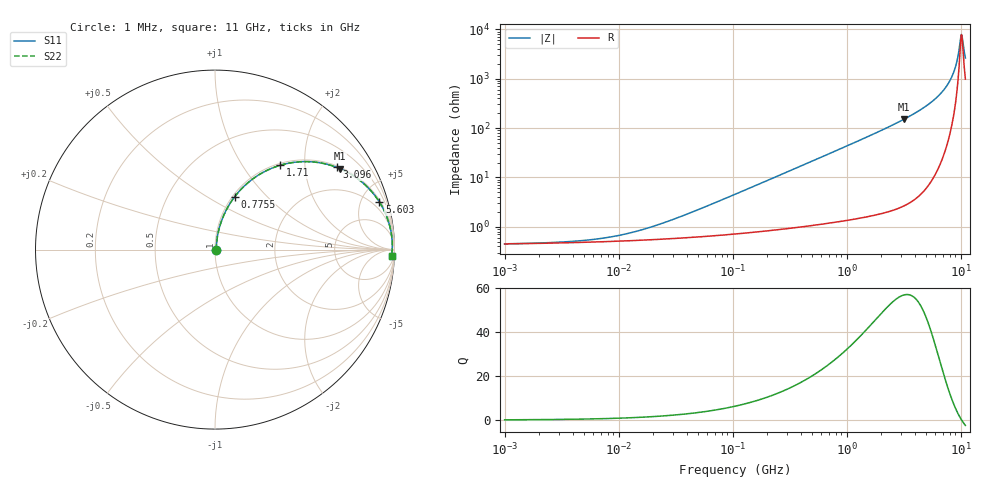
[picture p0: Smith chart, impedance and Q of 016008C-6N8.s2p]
# MHz S MA R 50
!Freq  MagS11  AngS11  MagS21  AngS21  MagS12  AngS12  MagS22  AngS22
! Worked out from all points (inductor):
!   801 points, 1 MHz to 11 GHz, reference 50 ohm
!   read as one part in series: L = 6.8 nH near 42.83 MHz
!   highest Q = 57.1 at 3.206 GHz (marker M1), where L = 7.55 nH
!   self-resonance near 10.14 GHz
!   S11 on the Smith chart (normalised r, x): 1 MHz: 1.01, +0.00; 775.5 MHz: 1.02, +0.67; 1.71 GHz: 1.03, +1.50; 3.096 GHz: 1.05, +2.92; 5.603 GHz: 1.18, +6.87; 11 GHz: 21, -49
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1  0.004485 5.4  0.9955 -0.0  0.9955 -0.0  0.004485 5.4
4.752622  0.005206 22.7  0.9952 -0.1  0.9952 -0.1  0.005206 22.7
10.48218  0.00677 40.9  0.9949 -0.3  0.9949 -0.3  0.00677 40.9
22.3262  0.01097 59.3  0.9944 -0.5  0.9944 -0.5  0.01097 59.3
104.8809  0.04501 78.4  0.9919 -2.5  0.9919 -2.5  0.04501 78.4
248.042  0.1049 79.3  0.9859 -6.0  0.9859 -6.0  0.1049 79.3
498.4592  0.2069 75.2  0.9682 -11.9  0.9682 -11.9  0.2069 75.2
775.5249  0.3129 69.7  0.9384 -18.2  0.9384 -18.2  0.3129 69.7
1165.217  0.4455 61.9  0.8828 -26.4  0.8828 -26.4  0.4455 61.9
1710.465  0.5948 52.2  0.7907 -36.5  0.7907 -36.5  0.5948 52.2
2341.592  0.7194 42.9  0.6809 -46.0  0.6809 -46.0  0.7194 42.9
3095.658  0.8179 34.1  0.5611 -54.9  0.5611 -54.9  0.8179 34.1
3205.591  0.8289 33.0  0.5451 -56.0  0.5451 -56.0  0.8289 33.0
4337.639  0.9085 23.6  0.4011 -65.3  0.4011 -65.3  0.9085 23.6
5602.627  0.9536 16.1  0.2777 -72.4  0.2777 -72.4  0.9536 16.1
6988.352  0.9771 10.0  0.1731 -77.4  0.1731 -77.4  0.9771 10.0
8224.304  0.986 5.6  0.09787 -79.0  0.09787 -79.0  0.986 5.6
9026.369  0.9881 3.1  0.05581 -76.1  0.05581 -76.1  0.9881 3.1
9792.087  0.9881 1.0  0.02131 -55.5  0.02131 -55.5  0.9881 1.0
10022.56  0.9878 0.4  0.01416 -30.3  0.01416 -30.3  0.9878 0.4
10378.49  0.9871 -0.5  0.01545 33.2  0.01545 33.2  0.9871 -0.5
11000  0.9853 -2.0  0.0376 66.0  0.0376 66.0  0.9853 -2.0
